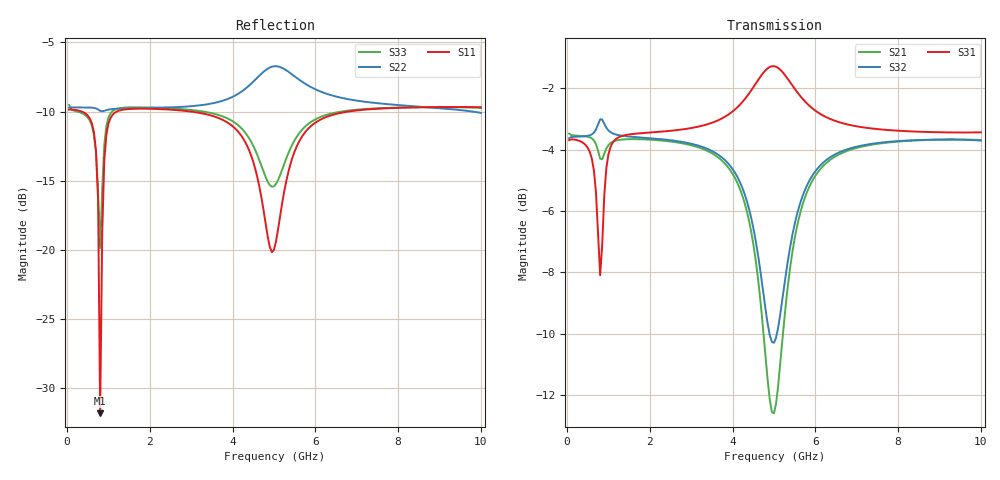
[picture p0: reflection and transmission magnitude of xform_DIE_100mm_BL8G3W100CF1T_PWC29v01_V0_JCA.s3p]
! Created Wed Dec 13 15:50:16 2017
# ghz S ma R 50
! 3 Port Network Data from SP1.SP block
! freq  magS11  angS11  magS12  angS12  magS13  angS13
!  magS21  angS21
!  magS22  angS22  magS23  angS23
!  magS31  angS31  magS32  angS32
!  magS33  angS33
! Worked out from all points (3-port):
!   200 points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, 50 MHz to 10 GHz, reference 50 ohm
!   strongest paths, dB at 50 MHz, 2.55 GHz, 5.05 GHz, 7.55 GHz, 10 GHz:
!     S31: -3.7, -3.4, -1.3, -3.3, -3.4
!     S32: -3.6, -3.7, -10.1, -3.8, -3.7
!     S21: -3.5, -3.7, -12.3, -3.8, -3.7
!   lowest |S11| = -31.8 dB at 800 MHz (marker M1), VSWR 1.05, Z = 49.7 + j2.54 ohm
!   |S11| at or under -10 dB: 358.9 MHz to 1.199 GHz (840.4 MHz wide, 108 % of centre); 2.997 GHz to 6.791 GHz (3.794 GHz wide, 77.5 % of centre)
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0.05  0.3213 -175.0  0.6702 -3.1  0.654 5.7
      0.6702 -3.1  0.3262 -174.3  0.6589 6.0
      0.654 5.7  0.6589 6.0  0.3339 -156.4
0.7  0.2271 138.0  0.6442 -4.5  0.5364 -10.9
     0.6442 -4.5  0.3247 173.8  0.6807 1.3
     0.5364 -10.9  0.6807 1.3  0.2246 157.3
0.75  0.1522 121.4  0.6281 -4.6  0.4601 -9.9
      0.6281 -4.6  0.322 173.2  0.6939 1.1
      0.4601 -9.9  0.6939 1.1  0.1613 155.7
0.8  0.02565 96.0  0.61 -3.5  0.394 1.7
     0.61 -3.5  0.3184 173.1  0.7072 -0.1
     0.394 1.7  0.7072 -0.1  0.1015 -174.4
0.9  0.2107 -126.6  0.6218 -0.1  0.5319 18.7
     0.6218 -0.1  0.3184 173.4  0.6953 -2.9
     0.5319 18.7  0.6953 -2.9  0.2401 -145.7
1.1  0.3079 -157.9  0.6499 -0.8  0.6476 11.1
     0.6499 -0.8  0.323 171.8  0.6709 -3.2
     0.6476 11.1  0.6709 -3.2  0.3176 -164.1
4.4  0.229 155.2  0.4825 -25.3  0.7794 8.1
     0.4825 -25.3  0.3927 76.6  0.5044 -20.4
     0.7794 8.1  0.5044 -20.4  0.2532 164.9
5.05  0.1074 -157.7  0.2431 11.8  0.8614 -0.6
      0.2431 11.8  0.4615 -11.1  0.3116 7.2
      0.8614 -0.6  0.3116 7.2  0.1731 -169.9
6.45  0.3087 -160.4  0.6133 15.9  0.7042 -5.3
      0.6133 15.9  0.36 -122.5  0.6186 12.6
      0.7042 -5.3  0.6186 12.6  0.3127 -167.0
10  0.328 -174.3  0.6544 3.8  0.6735 -0.9
    0.6544 3.8  0.3128 -167.5  0.6529 2.2
    0.6735 -0.9  0.6529 2.2  0.3261 -177.5
